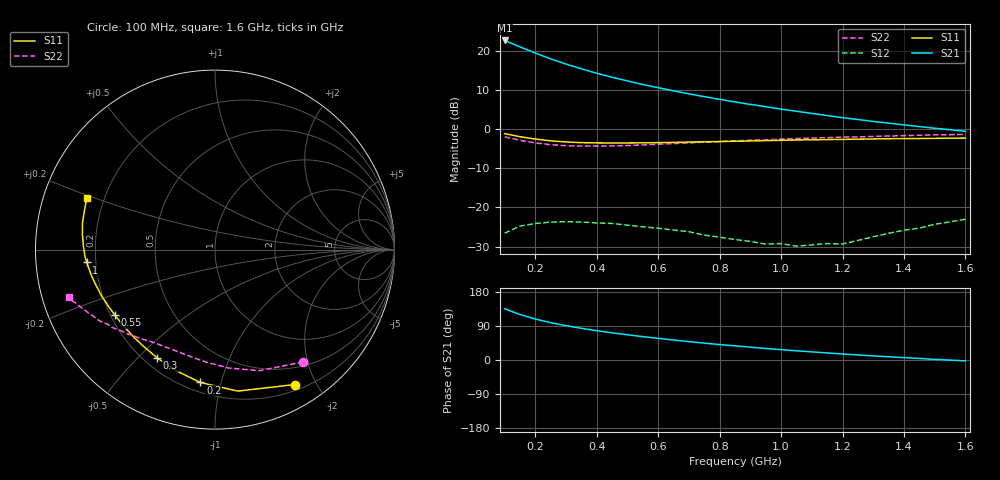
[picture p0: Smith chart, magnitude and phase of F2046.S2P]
! Date: Mon Aug 14 14:24:47 1995
# MHZ  S  MA  R  50.0000
!  POLYFET RF DEVICES
!  F2046
!  S PARAMETERS
!  VDS=28V, IDQ=800mA
! FREQ  S11MAG  S11ANG  S21MAG  S21ANG  S12MAG  S12ANG  S22MAG  S22ANG
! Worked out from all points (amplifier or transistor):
!   31 points, 100 MHz to 1.6 GHz, reference 50 ohm
!   highest |S21| = 22.6 dB at 100 MHz (marker M1)
!   |S21| within 3 dB of that: start of sweep to 193.1 MHz
!   unconditionally stable (mu >= 1): 821.7 MHz to 1.318 GHz
!   at 350 MHz: K = 0.32, MSG = 19.6 dB, |S12| = -23.8 dB
!   at 850 MHz: K = 1.05, MAG = 16.1 dB, |S12| = -28.2 dB
!   at 1.6 GHz: K = 0.51, MSG = 11.2 dB, |S12| = -23.0 dB
!   S11 on the Smith chart (normalised r, x): 100 MHz: 0.27, -1.72; 200 MHz: 0.26, -0.86; 300 MHz: 0.25, -0.57; 550 MHz: 0.22, -0.28; 1 GHz: 0.16, -0.05; 1.6 GHz: 0.14, +0.19
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100  0.8728 -59.5  13.51 135.3  0.04686 49.2  0.7962 -51.8
150  0.7985 -80.9  11.19 119.9  0.05775 36.0  0.7188 -69.7
200  0.7448 -96.2  9.327 108.1  0.06229 25.6  0.6648 -83.2
250  0.7072 -108.7  7.862 98.6  0.06485 17.7  0.631 -93.7
300  0.6837 -118.2  6.747 90.6  0.06576 12.4  0.6135 -101.6
350  0.6707 -126.1  5.864 83.6  0.06492 7.0  0.6059 -108.0
400  0.6654 -132.4  5.151 77.4  0.06328 3.7  0.6052 -113.5
450  0.6628 -137.9  4.578 71.8  0.06232 0.6  0.6102 -117.9
500  0.6642 -142.7  4.111 66.5  0.05923 -2.4  0.6166 -122.0
550  0.6662 -147.0  3.696 61.6  0.05661 -4.2  0.6268 -125.6
600  0.6708 -150.7  3.37 57.2  0.05421 -4.7  0.6403 -128.5
650  0.6754 -154.3  3.075 52.6  0.05138 -6.3  0.6529 -131.6
700  0.6825 -157.6  2.813 48.5  0.04894 -6.3  0.666 -134.4
800  0.6927 -163.5  2.395 40.7  0.04166 -3.8  0.691 -139.0
850  0.6991 -166.3  2.215 37.3  0.03893 -1.2  0.7066 -141.2
950  0.7113 -171.8  1.929 30.5  0.03403 4.5  0.7277 -145.1
1000  0.7181 -174.3  1.795 27.3  0.03449 11.6  0.7438 -146.9
1050  0.7252 -176.8  1.687 24.4  0.03199 18.9  0.7569 -148.4
1100  0.7287 -179.4  1.582 21.4  0.03324 22.8  0.7661 -150.2
1200  0.7373 175.9  1.397 15.8  0.03411 38.2  0.7876 -153.0
1350  0.7528 169.0  1.19 8.5  0.04668 50.9  0.8138 -156.8
1600  0.7673 158.0  0.9348 -2.4  0.07055 55.5  0.8567 -162.2
